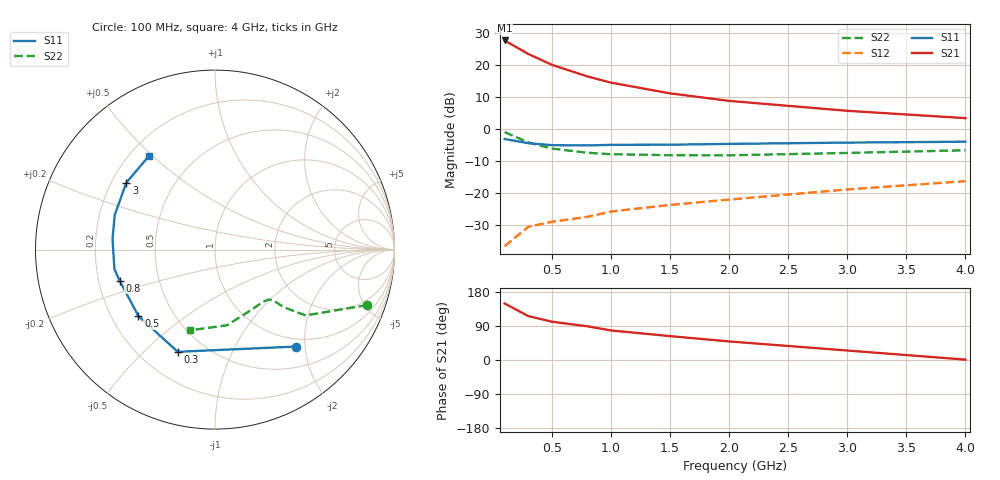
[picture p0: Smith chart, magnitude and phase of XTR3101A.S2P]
! HXTR-3101 Common Emitter
! Vce=10v  Ic= 10 mA
# ghz s ma r 50
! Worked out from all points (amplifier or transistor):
!   9 points, 100 MHz to 4 GHz, reference 50 ohm
!   highest |S21| = 27.7 dB at 100 MHz (marker M1)
!   |S21| within 3 dB of that: start of sweep to 242.8 MHz
!   unconditionally stable (mu >= 1): 1.212 GHz to 2.867 GHz
!   at 300 MHz: K = 0.44, MSG = 27.0 dB, |S12| = -30.5 dB
!   at 1 GHz: K = 0.94, MSG = 20.1 dB, |S12| = -25.7 dB
!   at 4 GHz: K = 0.84, MSG = 9.8 dB, |S12| = -16.2 dB
!   S11 on the Smith chart (normalised r, x): 100 MHz: 0.85, -1.83; 300 MHz: 0.36, -0.64; 500 MHz: 0.31, -0.34; 800 MHz: 0.29, -0.15; 3 GHz: 0.26, +0.31; 4 GHz: 0.28, +0.49
0.1  0.705 -50.0  24.27 149.0  0.015 60.0  0.903 -20.0
0.3  0.606 -110.0  14.96 116.0  0.03 43.0  0.624 -36.0
0.5  0.565 -139.0  10.12 101.0  0.036 41.0  0.499 -40.0
0.8  0.559 -162.0  6.68 89.0  0.043 43.0  0.43 -41.0
1  0.571 -169.0  5.33 78.0  0.052 44.0  0.408 -43.0
1.5  0.574 174.0  3.63 63.0  0.066 48.0  0.394 -48.0
2  0.591 161.0  2.77 49.0  0.08 48.0  0.392 -57.0
3  0.619 143.0  1.94 25.0  0.115 45.0  0.427 -81.0
4  0.639 125.0  1.49 1.0  0.155 39.0  0.47 -107.0
